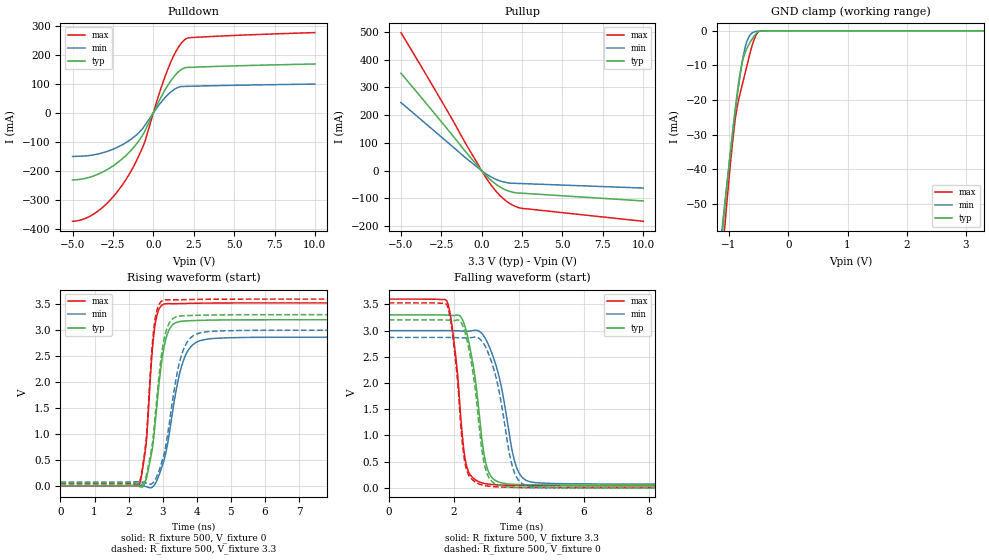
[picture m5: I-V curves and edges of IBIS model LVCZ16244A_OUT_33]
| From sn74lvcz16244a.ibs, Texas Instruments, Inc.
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[Model]   LVCZ16244A_OUT_33
Model_type  3-state
Enable   Active-Low
Vref =   0
Rref =   500
Cref =   50p
Vmeas =   1.5
| variable   typ   min   max
C_comp   6.56pF   5.68pF   7.78pF
| C_pullup   7.85pF   7.04pF   8.62pF
| C_pulldown   10.79pF   6.80pF   16.81pF
| C_tri-state   6.56pF   5.68pF   7.78pF
[Temperature Range]   40   100   -40
| Ambient temperature   25   85   -40
[Voltage range]   3.3   3   3.6
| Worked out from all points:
|   slope of the pulldown table from 0 to 0.495 V, typ, clamps not added: 8.8 ohm
|   slope of the pullup table from 0 to 0.495 V, typ, clamps not added: 16.5 ohm
|   GND clamp passes 1 mA (typ) near -0.55 V on its own axis
|   rising waveform, R_fixture 500, V_fixture 0: 20-80 % time 333ps typ, 479ps min, 229ps max; typ from 0 V to 3.2 V
|   falling waveform, R_fixture 500, V_fixture 3.3: 20-80 % time 411ps typ, 556ps min, 315ps max; typ from 3.3 V to 0.054 V
|   rising waveform, R_fixture 500, V_fixture 3.3: 20-80 % time 324ps typ, 452ps min, 225ps max; typ from 0.054 V to 3.3 V
|   falling waveform, R_fixture 500, V_fixture 0: 20-80 % time 394ps typ, 522ps min, 308ps max; typ from 3.2 V to 0 V
[GND Clamp]
| LVCZ16244A_OUT_33
|   Voltage   I(typ)   I(min)   I(max)
-5V       -857.7mA   -781.6mA   -988.1mA
-1.13V    -61.4mA    -59.12mA   -68.35mA
-1.1V     -56.08mA   -54.28mA   -62.24mA
-1.07V    -50.82mA   -49.5mA    -56.22mA
-910mV    -24.63mA   -25.39mA   -27.58mA
-865mV    -18.28mA   -19.26mA   -22.25mA
-800mV    -10.93mA   -11.35mA   -17.15mA
-740mV    -6.841mA   -5.661mA   -13.03mA
-685mV    -4.623mA   -2.44mA    -9.179mA
-585mV    -1.744mA   -371.7uA   -2.908mA
-495mV    -164.2uA   -98.78uA   -161.7uA
3.3V      12.36pA    55.94nA    5.986pA
[Pulldown]
| LVCZ16244A_OUT_33
|   Voltage   I(typ)   I(min)   I(max)
-5V       -231.6mA   -150.6mA   -374.6mA
-4.145V   -225.5mA   -148.5mA   -363.1mA
-3.275V   -208.1mA   -140mA     -332.8mA
-2.405V   -179.6mA   -123.3mA   -284.3mA
-1.585V   -141.2mA   -98.9mA    -220.5mA
-565mV    -67.24mA   -46.66mA   -105.9mA
370mV     42.84mA    28.84mA    67.73mA
995mV     103.8mA    67.97mA    164.5mA
1.49V     138.6mA    87.13mA    221.3mA
1.945V    155.7mA    91.51mA    253mA
2.85V     158.7mA    92.82mA    261.8mA
10V       169mA      99.65mA    277.6mA
[Pullup]
| LVCZ16244A_OUT_33
|   Voltage   I(typ)   I(min)   I(max)
-5V       351.5mA    245.5mA    497.7mA
-2.68V    189.3mA    130.6mA    270.7mA
-965mV    66.11mA    45mA       95.21mA
165mV     -10.82mA   -7.186mA   -15.94mA
830mV     -46.35mA   -29.7mA    -69.97mA
1.495V    -69.31mA   -42.29mA   -108.1mA
2.005V    -78.43mA   -45.26mA   -126.6mA
2.52V     -81.02mA   -46.38mA   -135.8mA
10V       -108.8mA   -62.36mA   -182.1mA
[Ramp]
| LVCZ16244A_OUT_33
| variable   typ   min   max
dV/dt_r   1.94/3.43E-10   1.74/4.91E-10   2.12/2.32E-10
dV/dt_f   1.95/4.15E-10   1.76/5.62E-10   2.14/3.18E-10
R_load = 500
[Rising Waveform]
| LVCZ16244A_OUT_33
R_fixture =   500
C_fixture =   0
L_fixture =   0
V_fixture =   0
V_fixture_min = 0
V_fixture_max = 0
|   Time   V(typ)   V(min)   V(max)
0s        81.93pV    2.924nV    53.66pV
2.305ns   -14.64mV   6.993mV    2.302mV
2.515ns   128.7mV    -18.18mV   816.7mV
2.67ns    620.4mV    -36.56mV   2.404V
2.77ns    1.149V     28.97mV    3.079V
3.065ns   2.756V     558.7mV    3.509V
3.27ns    3.09V      1.34V      3.512V
3.605ns   3.176V     2.409V     3.515V
4.28ns    3.193V     2.826V     3.524V
24.99ns   3.202V     2.866V     3.527V
[Falling Waveform]
| LVCZ16244A_OUT_33
R_fixture =   500
C_fixture =   0
L_fixture =   0
V_fixture =   3.3
V_fixture_min = 3
V_fixture_max = 3.6
|   Time   V(typ)   V(min)   V(max)
0s        3.3V       3V         3.6V
1.785ns   3.296V     3V         3.565V
2ns       3.288V     2.998V     2.822V
2.365ns   3.03V      2.988V     494mV
2.65ns    2.124V     3.007V     159.5mV
2.915ns   698.6mV    2.902V     87.75mV
3.375ns   113.1mV    2.164V     55.79mV
3.91ns    64.34mV    425.3mV    46.51mV
4.39ns    58.21mV    109.9mV    43.3mV
24.99ns   53.73mV    71.45mV    37.28mV
[Rising Waveform]
| LVCZ16244A_OUT_33
R_fixture =   500
C_fixture =   0
L_fixture =   0
V_fixture =   3.3
V_fixture_min = 3
V_fixture_max = 3.6
|   Time   V(typ)   V(min)   V(max)
0s        53.63mV    71.4mV     37.14mV
2.305ns   38.78mV    78.15mV    40.01mV
2.515ns   186.7mV    52.7mV     887.4mV
2.665ns   685.8mV    34.43mV    2.476V
2.765ns   1.242V     99.42mV    3.164V
2.935ns   2.369V     374.5mV    3.54V
3.055ns   2.868V     655.7mV    3.585V
3.565ns   3.276V     2.545V     3.589V
4.19ns    3.291V     2.962V     3.596V
24.99ns   3.3V       3V         3.6V
[Falling Waveform]
| LVCZ16244A_OUT_33
R_fixture =   500
C_fixture =   0
L_fixture =   0
V_fixture =   0
V_fixture_min = 0
V_fixture_max = 0
|   Time   V(typ)   V(min)   V(max)
0s        3.204V     2.87V      3.529V
1.785ns   3.2V       2.87V      3.493V
1.995ns   3.193V     2.868V     2.753V
2.35ns    2.953V     2.86V      454.8mV
2.615ns   2.089V     2.873V     130.7mV
2.91ns    543mV      2.759V     48.36mV
3.33ns    60.49mV    2.025V     18.97mV
3.82ns    10.89mV    368.5mV    9.807mV
4.305ns   4.138mV    32.9mV     6.316mV
24.99ns   108.9uV    50.21uV    130.8uV
